PROGRAM MAIN_CM
VAR CONSTANT														 
	cInitCrest 		: ST_CM_CrestFactor_InitPars := ( nChannels := cChannels, nBufferLength  := cBufferLength );									 
END_VAR
VAR		
	fbCrest				: FB_CMA_CrestFactor := (stInitPars := cInitCrest, nOwnID:= eID_Crest, aDestIDs:= [eID_Sink]);		// Initialize crest
	fbErrHist			: FB_HRErrHist; // error monitoring
END_VAR

// Call CrestFactor to calculate
fbCrest.Call();
IF fbCrest.bError THEN
	fbErrHist.AddError(bErr:=TRUE, hrErrCode:=fbCrest.hrErrorCode, sErrSource:='MAIN_CM.fbCrest'); // error monitoring
	//ToDo: if error
END_IF

END_PROGRAM
